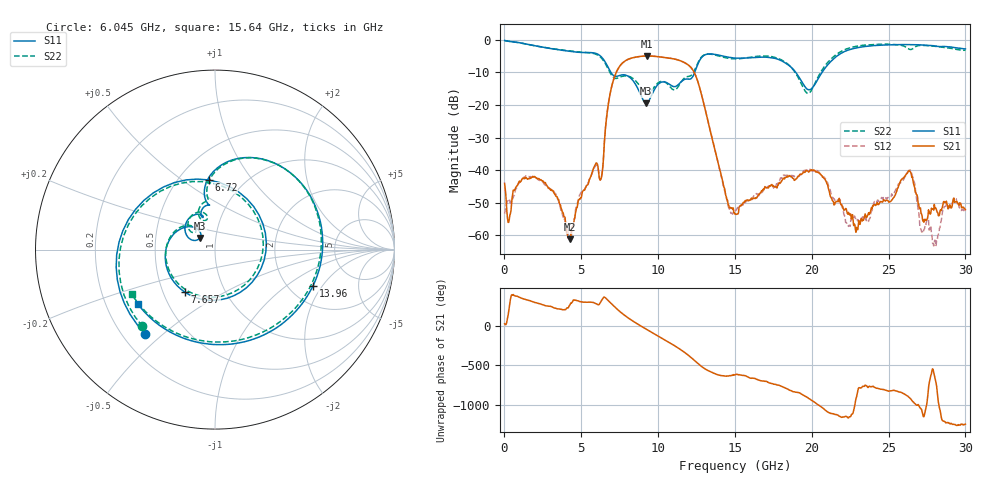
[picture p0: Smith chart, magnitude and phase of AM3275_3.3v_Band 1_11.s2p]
!Keysight Technologies,N5245B,MY58422270,A.16.20.02
!Date: Thursday, March 27, 2025 01:46:57
!Correction: S11(C  2-Port  )
!S21(C  2-Port  )
!S12(C  2-Port  )
!S22(C  2-Port  )
!S2P File: Measurements: S11, S21, S12, S22:
# Hz S  dB  R 50
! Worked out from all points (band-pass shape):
!   801 points, 10 MHz to 30 GHz, reference 50 ohm
!   highest |S21| = -4.94 dB at 9.269 GHz (marker M1); lowest = -61.2 dB at 4.284 GHz (marker M2)
!   |S21| within 3 dB of the highest: 7.525 GHz to 12.02 GHz (4.498 GHz wide, 46 % of centre)
!   lowest |S11| = -19.4 dB at 9.232 GHz (marker M3), VSWR 1.24, Z = 41.9 + j5.46 ohm
!   |S11| at or under -10 dB: 6.929 GHz to 12.38 GHz (5.451 GHz wide, 56.5 % of centre); 18.97 GHz to 20.66 GHz (1.699 GHz wide, 8.58 % of centre)
!   |S22| runs from -16.7 to -0.2 dB; largest |S21 - S12| = 0.005
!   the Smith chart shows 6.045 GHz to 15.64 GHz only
!   S11 on the Smith chart (normalised r, x): 6.045 GHz: 0.29, -0.44; 6.72 GHz: 0.69, +0.64; 7.657 GHz: 0.65, -0.34; 13.96 GHz: 2.67, -1.64; 15.64 GHz: 0.34, -0.28
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1e7  -0.18 -5.1  -44.04 23.1  -53.34 37.8  -0.21 -5.9
1.022162e9  -0.91 -83.0  -43.67 -7.8  -43.50 -6.0  -0.94 -83.4
2.221762e9  -2.00 -164.8  -42.54 -81.7  -42.98 -84.1  -2.01 -165.7
4.283575e9  -3.52 65.4  -61.15 -92.2  -61.14 -74.5  -3.39 64.3
5.033325e9  -3.86 2.5  -47.57 -64.1  -46.52 -60.6  -3.78 1.0
6.045488e9  -4.32 -129.7  -38.11 -92.9  -38.60 -92.9  -4.60 -133.5
6.720262e9  -8.19 95.2  -21.05 -38.6  -20.97 -39.0  -8.65 91.3
7.65745e9  -10.74 -125.0  -7.21 153.6  -7.21 153.5  -11.19 -121.9
9.231925e9  -19.44 142.8  -4.94 -45.2  -4.94 -45.2  -16.61 136.3
9.269412e9  -19.39 145.4  -4.94 -49.4  -4.93 -49.4  -16.66 137.3
1.001916e10  -13.55 142.6  -5.16 -132.3  -5.15 -132.3  -13.13 131.3
1.114379e10  -14.29 111.4  -5.96 99.4  -5.95 99.3  -15.24 111.2
1.395535e10  -4.70 -20.3  -38.58 98.7  -38.77 100.2  -4.95 -24.6
1.5005e10  -5.59 -100.1  -53.48 102.7  -52.82 105.2  -5.81 -106.6
1.564229e10  -5.59 -145.0  -49.54 93.1  -50.00 86.5  -5.58 -151.6
1.762912e10  -5.68 101.6  -45.00 -17.2  -45.26 -17.0  -5.40 98.7
2.002832e10  -14.78 -106.7  -39.95 138.1  -40.06 139.7  -15.03 -119.3
2.235255e10  -3.15 113.2  -53.48 -75.6  -56.65 -70.0  -2.63 109.8
2.501416e10  -1.54 39.1  -49.79 -102.7  -48.31 -87.9  -1.33 36.3
2.64012e10  -1.46 6.0  -40.36 167.7  -39.91 169.7  -2.95 4.6
2.801316e10  -1.86 -37.7  -51.57 72.2  -61.43 -130.9  -1.96 -38.8
3e10  -2.77 -108.7  -52.10 -156.1  -52.41 172.5  -3.18 -110.6
